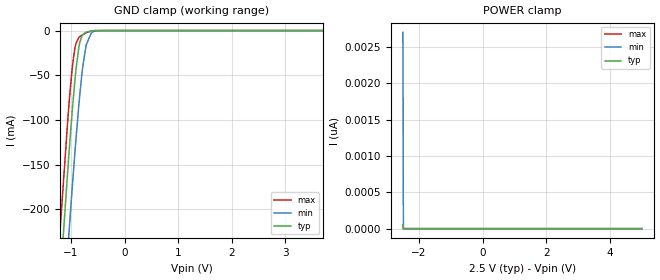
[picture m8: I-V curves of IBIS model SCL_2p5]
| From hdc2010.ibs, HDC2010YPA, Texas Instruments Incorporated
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[Model]   SCL_2p5
Model_type   Input
Vinl = 0.75
Vinh = 1.75
|   typ   min   max
|   (nom PVT)   (slow PVT)   (fast PVT)
C_comp   0.671p   0.651p   0.685p
[Model spec]
|subparameter
Vinl   0.75   0.675   0.825
Vinh   1.75   1.575   1.925
[Voltage Range]   2.5   2.25   2.75
[Temperature Range]   27   125   -40
[Power Clamp Reference]   2.5   2.25   2.75
[GND Clamp Reference]   0   0   0
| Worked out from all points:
|   GND clamp passes 1 mA (typ) near -0.66 V on its own axis
[GND Clamp]
|   Voltage   I(typ)   I(min)   I(max)
-2.5V     -1.528A    -1.611A    -1.475A
-1.218V   -295.6mA   -386.5mA   -237mA
-1.052V   -151.4mA   -240.8mA   -95.57mA
-1.038V   -139.1mA   -228mA     -84.07mA
-970mV    -86.53mA   -172mA     -39.18mA
-925mV    -55.67mA   -136.5mA   -19.66mA
-850mV    -18.28mA   -82.37mA   -7.68mA
-775mV    -4.458mA   -38.81mA   -4.512mA
-715mV    -1.826mA   -16.17mA   -2.449mA
-617.5mV  -350.5uA   -2.47mA    -388.3uA
-475mV    -11.27uA   -123.5uA   -4.168uA
5V        0A         0A         0A
[POWER Clamp]
|   Voltage   I(typ)   I(min)   I(max)
-2.5V     53.73pA    2.702nA    46.76pA
-2.485V   0A         0A         0A
-2.478V   0A         0A         0A
5V        0A         0A         0A
